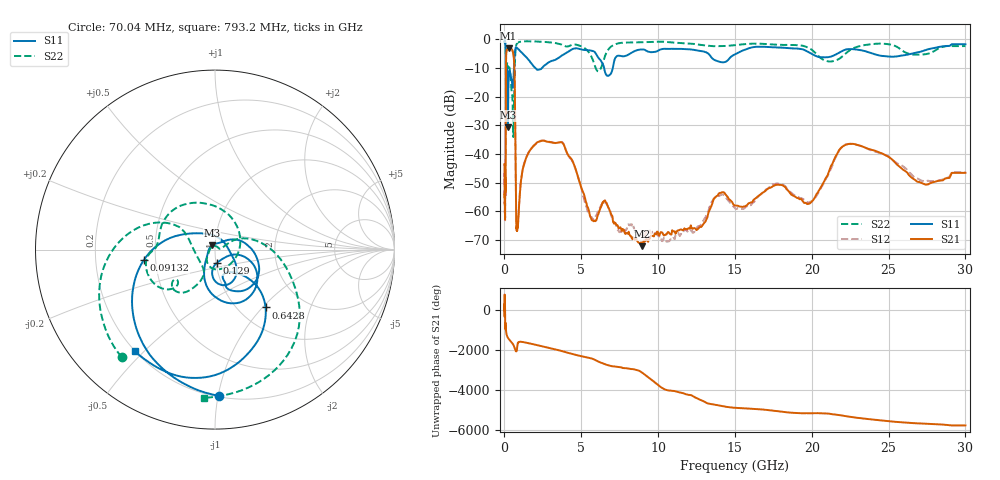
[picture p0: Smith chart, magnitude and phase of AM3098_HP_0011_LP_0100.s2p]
! Date/Time: Thu, Feb 28, 2019 8:34 AM
! Network Analyzer: Agilent Technologies E8364B Rev: A.07.50.67
! Sweep from 0.010 to 30.000 GHz, 1601 Points, Sweep Type: LOG
! Power Supply: 5.022 V, 0.002 A
# Hz S DB R 50
!freq MagS11 AngS11 MagS21 AngS21 MagS12 AngS12 MagS22 AngS22
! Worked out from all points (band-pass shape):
!   1601 points, 10 MHz to 30 GHz, reference 50 ohm
!   highest |S21| = -3.04 dB at 266.5 MHz (marker M1); lowest = -72.2 dB at 8.982 GHz (marker M2)
!   |S21| within 3 dB of the highest: 107.5 MHz to 601.6 MHz (494.1 MHz wide, 139 % of centre)
!   lowest |S11| = -30.6 dB at 228.2 MHz (marker M3), VSWR 1.06, Z = 48.2 + j2.29 ohm
!   |S11| at or under -10 dB: 176.2 MHz to 619.1 MHz (442.9 MHz wide, 111 % of centre); 2.013 GHz to 2.43 GHz (417.6 MHz wide, 18.8 % of centre); 6.489 GHz to 7.049 GHz (560 MHz wide, 8.27 % of centre)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
!   |S22| runs from -34.1 to -0.5 dB; largest |S21 - S12| = 0.011
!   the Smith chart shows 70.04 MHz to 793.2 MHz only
!   S11 on the Smith chart (normalised r, x): 70.04 MHz: 0.21, -1.00; 91.32 MHz: 0.43, -0.06; 129 MHz: 1.01, -0.15; 642.8 MHz: 1.32, -1.04; 793.2 MHz: 0.20, -0.47
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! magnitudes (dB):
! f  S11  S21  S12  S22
! 10 MHz  -0.3  -43.4  -45.5  -0.5
! 38.04 MHz  -0.5  -61.8  -60.2  -0.8
! 48.61 MHz  -0.8  -49.1  -51.4  -1.2
! 70.04 MHz  -1.8  -52.1  -53.6  -2.0
! 91.32 MHz  -7.9  -19.9  -19.9  -9.4
! 100.9 MHz  -23.7  -8.1  -8.1  -17.2
! 129 MHz  -22.7  -4.1  -4.1  -11.0
! 144.7 MHz  -14.2  -3.7  -3.6  -10.3
! 185.8 MHz  -11.2  -3.5  -3.5  -8.1
! 228.2 MHz  -30.6  -3.1  -3.1  -9.6
! 266.5 MHz  -14.8  -3.0  -3.0  -9.9
! 550.5 MHz  -16.8  -4.4  -4.3  -30.0
! 642.8 MHz  -7.4  -9.8  -9.7  -16.4
! 793.2 MHz  -2.8  -66.0  -67.0  -1.6
! 2.084 GHz  -10.4  -36.2  -36.2  -0.7
! 3.779 GHz  -5.5  -36.2  -36.0  -1.9
! 5.612 GHz  -3.9  -62.2  -62.0  -5.5
! 7.926 GHz  -5.7  -67.6  -66.2  -1.1
! 8.982 GHz  -3.5  -72.2  -68.4  -1.0
! 19.7 GHz  -4.2  -57.5  -56.9  -2.7
! 22.67 GHz  -3.4  -36.5  -36.5  -3.2
! 30 GHz  -1.7  -46.6  -46.4  -2.3
